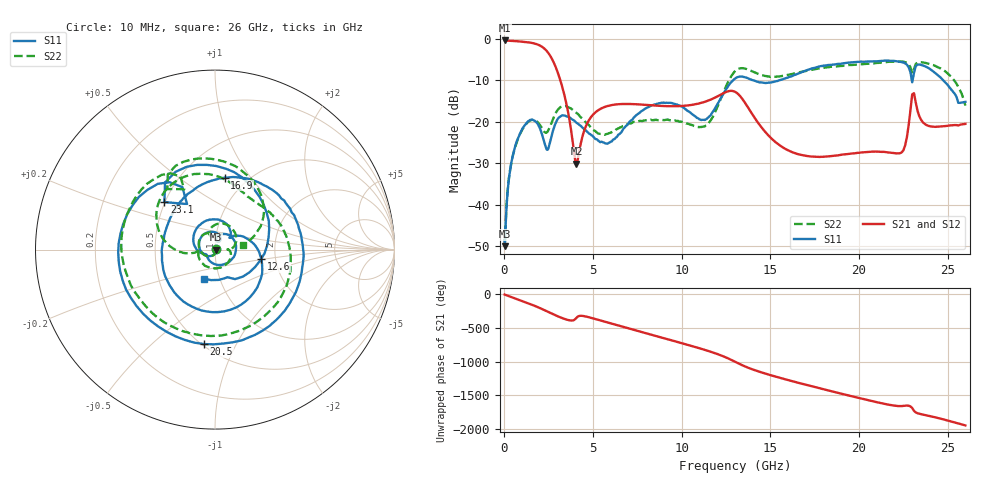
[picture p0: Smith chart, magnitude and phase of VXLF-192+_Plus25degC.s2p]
! Mini-Circuits
! S2P DATA File Format
! Type: LOW PASS FILTER
! Model: VXLF-192+
! All S Parameters are in dB deg format
! TEST CONDITIONS: INPUT POWER = 0 dBm @ Temperature = +25deg C
# MHz S dB R 50
!Frequency  S11 dB  S11 DEG  S21 dB  S21 DEG  S12 dB  S12 DEG  S22 dB  S22 DEG
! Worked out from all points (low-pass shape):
!   1260 points, 10 MHz to 26 GHz, reference 50 ohm
!   highest |S21| = -0.46 dB at 10 MHz (marker M1); lowest = -30.1 dB at 4.06 GHz (marker M2)
!   |S21| within 3 dB of the highest: start of sweep to 2.473 GHz
!   lowest |S11| = -49.9 dB at 30 MHz (marker M3), VSWR 1.01, Z = 50.3 - j0.0891 ohm
!   |S11| at or under -10 dB: start of sweep to 12.9 GHz; 13.99 GHz to 15.54 GHz (1.546 GHz wide, 10.5 % of centre); 24.74 GHz to end of sweep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
!   |S22| runs from -49.7 to -5.5 dB; largest |S21 - S12| = 0.0035
!   S11 on the Smith chart (normalised r, x): 10 MHz: 1.01, +0.00; 12.6 GHz: 1.68, -0.19; 16.9 GHz: 0.79, +0.76; 20.5 GHz: 0.51, -0.75; 23.1 GHz: 0.50, +0.31; 26 GHz: 0.85, -0.28
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10  -48.42 30.2  -0.46 -1.0  -0.46 -1.0  -49.72 16.3
30  -49.93 -16.1  -0.47 -3.0  -0.47 -3.0  -48.36 -15.1
310  -31.92 -96.0  -0.55 -29.9  -0.55 -29.9  -31.81 -94.7
890  -22.73 -165.7  -0.70 -85.8  -0.70 -85.8  -22.82 -161.2
1700  -19.77 105.9  -1.20 -168.6  -1.20 -168.6  -19.62 123.4
2410  -26.76 71.2  -3.12 108.3  -3.12 108.2  -22.52 106.3
2960  -19.67 56.8  -7.62 40.9  -7.62 40.9  -17.43 92.6
4060  -20.24 -55.7  -30.08 11.7  -30.08 11.7  -17.87 22.6
4350  -21.20 -78.8  -24.41 42.6  -24.40 42.6  -19.06 11.4
8680  -15.62 113.4  -16.16 91.6  -16.15 91.6  -19.65 -95.6
11300  -19.60 38.8  -15.23 -104.6  -15.20 -104.7  -21.15 -178.5
12600  -11.57 -11.6  -12.71 130.3  -12.75 129.8  -10.55 168.2
13050  -9.51 -59.4  -12.91 73.0  -13.03 72.7  -7.68 138.4
14350  -10.51 -171.3  -20.53 -67.8  -20.55 -66.9  -8.55 73.3
16900  -7.85 82.3  -28.12 102.5  -28.03 102.9  -7.88 11.3
17350  -7.17 64.0  -28.38 71.8  -28.31 72.1  -7.52 -3.4
19000  -6.04 -14.6  -27.95 -36.7  -27.96 -36.8  -6.60 -66.5
20500  -5.51 -96.7  -27.28 -132.8  -27.28 -132.4  -6.07 -134.1
21700  -5.32 -166.9  -27.41 157.8  -27.33 157.7  -5.59 171.4
23100  -8.25 136.8  -13.15 67.5  -13.10 67.5  -7.34 128.2
24600  -9.37 28.2  -21.13 -48.8  -21.19 -49.3  -7.19 60.8
26000  -15.23 -109.8  -20.53 -150.0  -20.56 -149.6  -16.12 10.1
